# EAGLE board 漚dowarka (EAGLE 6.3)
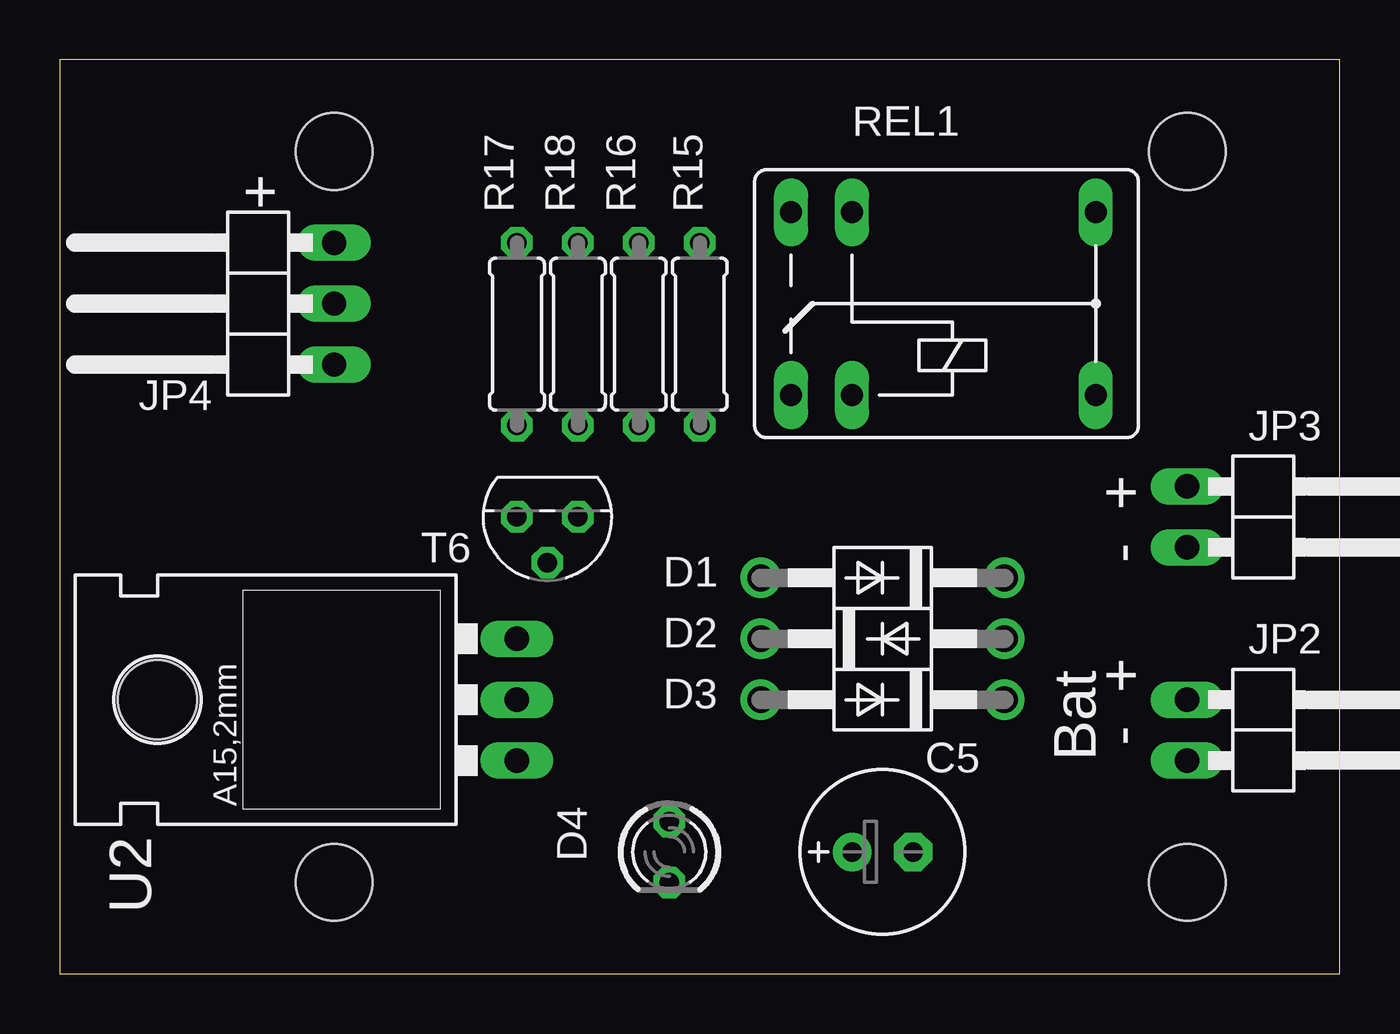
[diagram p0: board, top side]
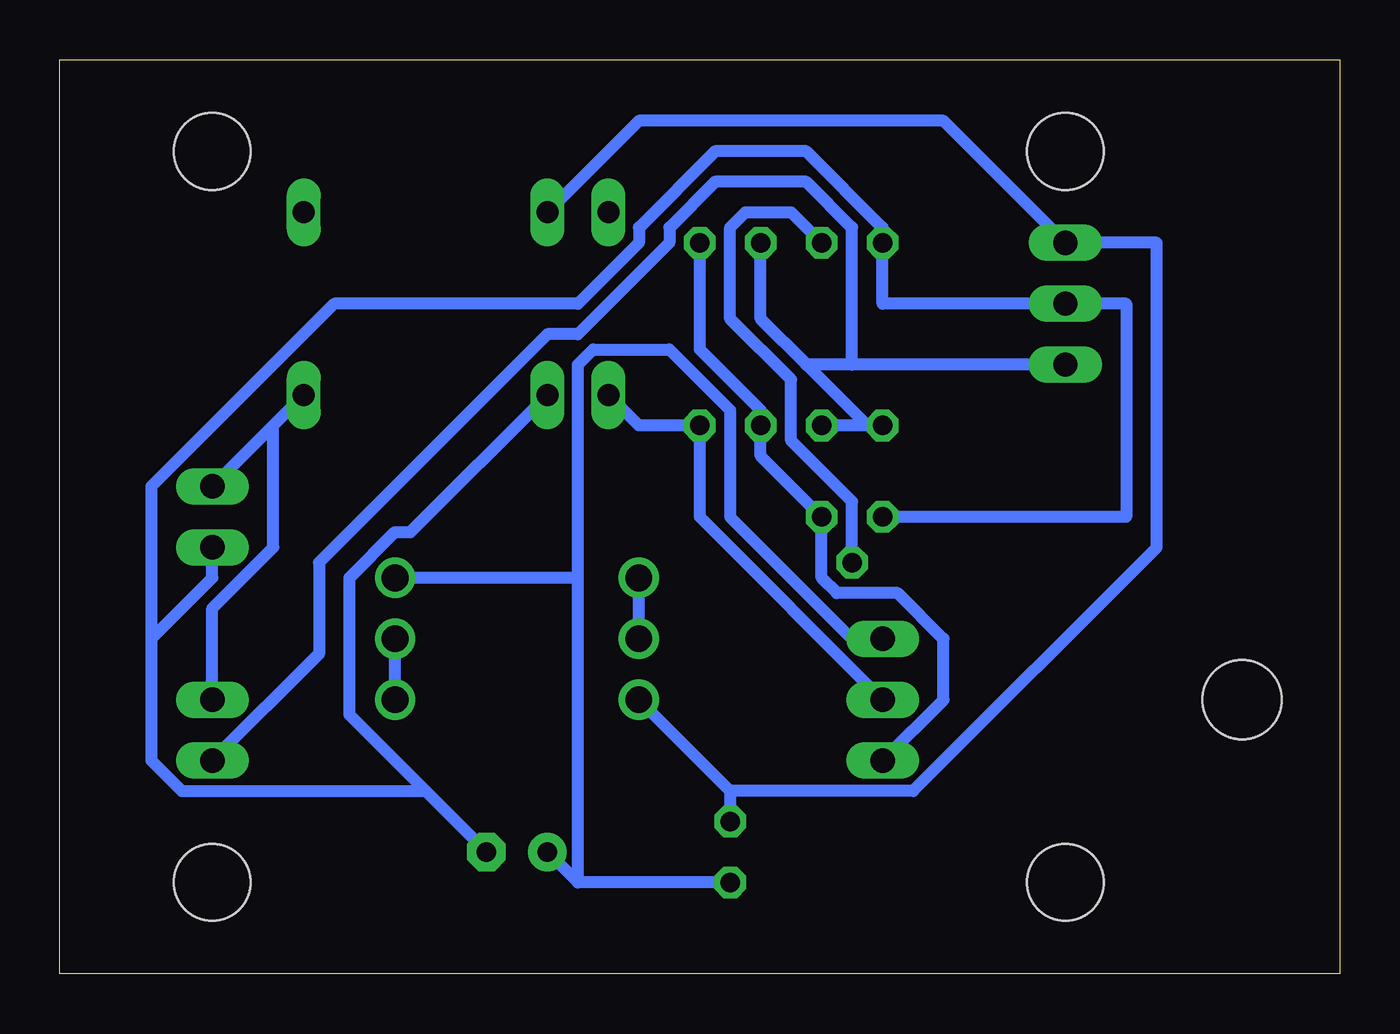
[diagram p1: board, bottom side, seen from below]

Size 53.34 x 38.1 mm. Coordinates in mm from the lower left corner, seen from the top.
Outline: 0,0 53.34,0 53.34,38.1 0,38.1 0,0
Copper layers (1*16): Top 0.035mm / dielectric 1.5mm / Bottom 0.035mm
Design rules "default *": minimum track width 20mil, minimum drill 24mil, track to track 8mil, track to pad 8mil, pad to pad 8mil, via to via 8mil, smd to smd 8mil, copper to edge 40mil, drill to drill 8mil, minimum pad ring 10mil, minimum via ring 8mil, stop-mask expansion 4mil, vias tented up to drill 0mil, thermal gap 10mil
Holes 3.2 mm at 11.43,34.29 11.43,3.81 46.99,34.29 46.99,3.81

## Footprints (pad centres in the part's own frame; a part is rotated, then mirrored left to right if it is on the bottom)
E2,5-7 = drill 0.813 pad 1.6: + -1.27,0 | drill 0.813 pad 1.6 octagon: - 1.27,0
DO41-10 = drill 1.118: A 5.08,0; C -5.08,0
LED3MM = drill 0.813 octagon: A -1.27,0; K 1.27,0
1X02/90 = drill 1.016 long: 1 -1.27,-3.81; 2 1.27,-3.81
1X03/90 = drill 1.016 long: 1 -2.54,-3.81; 2 0,-3.81; 3 2.54,-3.81
0207/7 = drill 0.813 octagon: 1 -3.81,0; 2 3.81,0
FRS1B = drill 0.914 long: 1 0,3.81; 2 0,-3.81; O -2.54,-3.81; P 10.16,3.81; P@ 10.16,-3.81; S -2.54,3.81
TO92 = drill 0.813 octagon: 1 1.27,0; 2 0,1.905; 3 -1.27,0
317TL = drill 1.016 long: 1 -2.54,-3.81; 2 0,-3.81; 3 2.54,-3.81 | hole 3.302: 0,11.176

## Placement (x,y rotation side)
C5  100uF  [E2,5-7]  34.29,5.08 0 top
D1  1N4004  [DO41-10]  34.29,16.51 180 top
D2  1N4004  [DO41-10]  34.29,13.97 0 top
D3  1N4004  [DO41-10]  34.29,11.43 180 top
D4  [LED3MM]  25.4,5.08 270 top
JP2  Bateria  [1X02/90]  50.8,10.16 270 top
JP3  Minutnik  [1X02/90]  50.8,19.05 270 top
JP4  Zasilanie  [1X03/90]  7.62,27.94 90 top
R15  240R  [0207/7]  26.67,26.67 270 top
R16  610R  [0207/7]  24.13,26.67 90 top
R17  4.7R  [0207/7]  19.05,26.67 90 top
R18  100R  [0207/7]  21.59,26.67 90 top
REL1  HFD41  [FRS1B]  33.02,27.94 0 top
T6  BC548  [TO92]  20.32,19.05 180 top
U2  LM317  [317TL]  15.24,11.43 90 top

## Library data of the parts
C5 R15-R18 = rcl
D1-D3 = diode
D4 = led
JP2-JP4 = pinhead
REL1 = relay
T6 = transistor-neu-to92
U2 = v-reg

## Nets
N$1: D2.A D3.C
N$2: C5.+ D1.C D4.K U2.3
N$3: R15.2 REL1.O U2.2
N$4: D3.A D4.A JP4.3 REL1.1
N$5: R15.1 R16.1 T6.3 U2.1
N$6: JP2.2 JP4.1 R16.2 R17.1 R18.1
N$7: R18.2 T6.2
N$8: C5.- JP3.2 JP4.2 R17.2 REL1.2 T6.1
N$9: D1.A D2.C
N$10: JP2.1 JP3.1 REL1.P@

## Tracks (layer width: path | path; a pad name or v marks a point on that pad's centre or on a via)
N$1
  Bottom 0.508: D3.C D2.A
N$2
  Bottom 0.508: D4.K 31.75,3.81 | 31.75,3.81 C5.+ | U2.3 20.32,13.97 25.4,19.05 25.4,23.5 27.94,26.04 31.11,26.04 31.75,25.4 31.75,16.51 | 31.75,3.81 31.75,16.51 | 31.75,16.51 D1.C
N$3
  Bottom 0.508: REL1.O 29.21,22.86 R15.2 26.67,19.05 U2.2
N$4
  Bottom 0.508: 25.4,7.62 D4.A | 25.4,7.62 D3.A | REL1.1 29.21,35.56 16.51,35.56 JP4.3 7.62,30.48 7.62,17.78 17.78,7.62 25.4,7.62
N$5
  Bottom 0.508: R15.1 26.67,26.04 24.13,23.5 R16.1 24.13,21.59 T6.3 21.59,16.51 20.96,15.88 18.41,15.88 16.51,13.97 16.51,11.43 U2.1
N$6
  Bottom 0.508: 19.68,22.86 R18.1 | R16.2 24.13,27.3 22.23,25.4 | 22.23,25.4 19.68,22.86 | 19.68,22.86 R17.1 | 20.32,25.4 22.23,25.4 | JP4.1 20.32,25.4 | JP2.2 42.54,13.34 42.54,17.14 33.02,26.67 31.75,26.67 27.94,30.48 27.94,31.11 26.04,33.02 22.23,33.02 20.32,31.11 20.32,25.4
N$7
  Bottom 0.508: T6.2 20.32,19.68 22.86,22.23 22.86,24.77 25.4,27.3 25.4,31.11 24.77,31.75 22.86,31.75 R18.2
N$8
  Bottom 0.508: T6.1 8.89,19.05 8.89,27.94 JP4.2 19.05,27.94 R17.2 19.05,31.11 22.23,34.29 26.04,34.29 29.21,31.11 29.21,30.48 31.75,27.94 41.91,27.94 49.53,20.32 49.53,13.97 | REL1.2 38.73,18.41 39.37,18.41 41.27,16.51 41.27,10.79 38.1,7.62 | 38.1,7.62 C5.- | JP3.2 46.99,16.51 49.53,13.97 | 49.53,13.97 49.53,8.89 48.26,7.62 38.1,7.62
N$9
  Bottom 0.508: D2.C D1.A
N$10
  Bottom 0.508: 44.45,22.86 JP3.1 | 44.45,22.86 REL1.P@ | JP2.1 46.99,15.24 44.45,17.78 44.45,22.86

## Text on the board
tNames: + | - + | - + | Bat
